(* Logix 5000 Rung export; software revision 13.03 *)

TYPE BIS_M_Userparameter :
STRUCT
   CRC_16 : SINT;   // 00h=disable, 01h=enable
   Simultan : SINT;   // 00h=disable, 01h=enable
   Dynamic_Head1 : SINT;   // 00h=disable, 01h=enable
   Dynamic_Head2 : SINT;   // 00h=disable, 01h=enable
   Extra_Haed1 : SINT;   // 00h=disable, 01h=enable
   Extra_Head2 : SINT;   // 00h=disable, 01h=enable
   Extra_Adr_Head1 : INT;   // 0 - 8191
   Extra_Adr_Head2 : INT;   // 0 - 8191
   TypSN : SINT;   // 00h=disable, 01h=enable
   DTTyp : SINT;   // 00h=All types, 01h=BIS M-1xx, 02h=not valid, 03h=not valid
END_STRUCT
END_TYPE

VAR_GLOBAL   (* controller tags *)
   control_bism1_par3 : MESSAGE;   // Parameter 3 write - Dynamic1
        MessageParameters(MessageType := CIP Generic, RequestedLength := 1, ConnectedFlag := 2, ConnectionPath := BIS_M, ServiceCode := 16#0010, ObjectType := 16#0064, TargetObject := 1, AttributeNumber := 16#0003, LocalElement := Userparameter_write_BISM_1.Dynamic_Head1)
   state_bism1_par1 : MESSAGE;   // Parameter 1 read - CRC
        MessageParameters(MessageType := CIP Generic, ConnectedFlag := 2, ConnectionPath := BIS_M, ServiceCode := 16#000e, ObjectType := 16#0064, TargetObject := 1, AttributeNumber := 16#0001, DestinationTag := Userparameter_read_BISM_1.CRC_16)
   control_bism1_par2 : MESSAGE;   // Parameter 2 write - Simultan
        MessageParameters(MessageType := CIP Generic, RequestedLength := 1, ConnectedFlag := 2, ConnectionPath := BIS_M, ServiceCode := 16#0010, ObjectType := 16#0064, TargetObject := 1, AttributeNumber := 16#0002, LocalElement := Userparameter_write_BISM_1.Simultan)
   control_bism1_par4 : MESSAGE;   // Parameter 4 write - Dynamic2
        MessageParameters(MessageType := CIP Generic, RequestedLength := 1, ConnectedFlag := 2, ConnectionPath := BIS_M, ServiceCode := 16#0010, ObjectType := 16#0064, TargetObject := 1, AttributeNumber := 16#0004, LocalElement := Userparameter_write_BISM_1.Dynamic_Head2)
   control_bism1_par6 : MESSAGE;   // Parameter 6 write - Extra2
        MessageParameters(MessageType := CIP Generic, RequestedLength := 1, ConnectedFlag := 2, ConnectionPath := BIS_M, ServiceCode := 16#0010, ObjectType := 16#0064, TargetObject := 1, AttributeNumber := 16#0006, LocalElement := Userparameter_write_BISM_1.Extra_Head2)
   state_bism1_par4 : MESSAGE;   // Patameter 4 read - Dynamic2
        MessageParameters(MessageType := CIP Generic, ConnectedFlag := 2, ConnectionPath := BIS_M, ServiceCode := 16#000e, ObjectType := 16#0064, TargetObject := 1, AttributeNumber := 16#0004, DestinationTag := Userparameter_read_BISM_1.Dynamic_Head2)
   control_bism1_par9 : MESSAGE;   // Parameter 9 write - Typ SN
        MessageParameters(MessageType := CIP Generic, RequestedLength := 1, ConnectedFlag := 2, ConnectionPath := BIS_M, ServiceCode := 16#0010, ObjectType := 16#0064, TargetObject := 1, AttributeNumber := 16#0009, LocalElement := Userparameter_write_BISM_1.TypSN)
   state_bism1_parA : MESSAGE;   // Patameter 10 read - DTTyp
        MessageParameters(MessageType := CIP Generic, ConnectedFlag := 2, ConnectionPath := BIS_M, ServiceCode := 16#000e, ObjectType := 16#0064, TargetObject := 1, AttributeNumber := 16#000a, DestinationTag := Userparameter_read_BISM_1.DTTyp)
   state_bism1_par7 : MESSAGE;   // Patameter 7 read - Extra_Adr1
        MessageParameters(MessageType := CIP Generic, ConnectedFlag := 2, ConnectionPath := BIS_M, ServiceCode := 16#000e, ObjectType := 16#0064, TargetObject := 1, AttributeNumber := 16#0007, DestinationTag := Userparameter_read_BISM_1.Extra_Adr_Head1)
   state_bism1_par6 : MESSAGE;   // Patameter 6 read - Extra2
        MessageParameters(MessageType := CIP Generic, ConnectedFlag := 2, ConnectionPath := BIS_M, ServiceCode := 16#000e, ObjectType := 16#0064, TargetObject := 1, AttributeNumber := 16#0006, DestinationTag := Userparameter_read_BISM_1.Extra_Head2)
   control_bism1_par1 : MESSAGE;   // Parameter 1write - CRC
        MessageParameters(MessageType := CIP Generic, RequestedLength := 1, ConnectedFlag := 2, ConnectionPath := BIS_M, ServiceCode := 16#0010, ObjectType := 16#0064, TargetObject := 1, AttributeNumber := 16#0001, LocalElement := Userparameter_write_BISM_1.CRC_16)
   Userparameter_read_BISM_1 : BIS_M_Userparameter;
   state_bism1_par3 : MESSAGE;   // Parameter 3 read - Dynamic1
        MessageParameters(MessageType := CIP Generic, ConnectedFlag := 2, ConnectionPath := BIS_M, ServiceCode := 16#000e, ObjectType := 16#0064, TargetObject := 1, AttributeNumber := 16#0003, DestinationTag := Userparameter_read_BISM_1.Dynamic_Head1)
   state_bism1_par2 : MESSAGE;   // Parameter 2 read - Simultan
        MessageParameters(MessageType := CIP Generic, ConnectedFlag := 2, ConnectionPath := BIS_M, ServiceCode := 16#000e, ObjectType := 16#0064, TargetObject := 1, AttributeNumber := 16#0002, DestinationTag := Userparameter_read_BISM_1.Simultan)
   Userparameter_write_BISM_1 : BIS_M_Userparameter;
   state_bism1_par5 : MESSAGE;   // Patameter 5 read - Extra1
        MessageParameters(MessageType := CIP Generic, ConnectedFlag := 2, ConnectionPath := BIS_M, ServiceCode := 16#000e, ObjectType := 16#0064, TargetObject := 1, AttributeNumber := 16#0005, DestinationTag := Userparameter_read_BISM_1.Extra_Haed1)
   control_bism1_par5 : MESSAGE;   // Parameter 5 write - Extra1
        MessageParameters(MessageType := CIP Generic, RequestedLength := 1, ConnectedFlag := 2, ConnectionPath := BIS_M, ServiceCode := 16#0010, ObjectType := 16#0064, TargetObject := 1, AttributeNumber := 16#0005, LocalElement := Userparameter_write_BISM_1.Extra_Haed1)
   control_bism1_parA : MESSAGE;   // Parameter 10 write - DTTyp
        MessageParameters(MessageType := CIP Generic, RequestedLength := 1, ConnectedFlag := 2, ConnectionPath := BIS_M, ServiceCode := 16#0010, ObjectType := 16#0064, TargetObject := 1, AttributeNumber := 16#000a, LocalElement := Userparameter_write_BISM_1.DTTyp)
   control_bism1_par7 : MESSAGE;   // Parameter 7 write - Extra_Adr1
        MessageParameters(MessageType := CIP Generic, RequestedLength := 2, ConnectedFlag := 2, ConnectionPath := BIS_M, ServiceCode := 16#0010, ObjectType := 16#0064, TargetObject := 1, AttributeNumber := 16#0007, LocalElement := Userparameter_write_BISM_1.Extra_Adr_Head1)
   control_bism1_par8 : MESSAGE;   // Parameter 8 write - Extra_Adr2
        MessageParameters(MessageType := CIP Generic, RequestedLength := 2, ConnectedFlag := 2, ConnectionPath := BIS_M, ServiceCode := 16#0010, ObjectType := 16#0064, TargetObject := 1, AttributeNumber := 16#0008, LocalElement := Userparameter_write_BISM_1.Extra_Adr_Head2)
   state_bism1_par9 : MESSAGE;   // Patameter 9 read - TypSN
        MessageParameters(MessageType := CIP Generic, ConnectedFlag := 2, ConnectionPath := BIS_M, ServiceCode := 16#000e, ObjectType := 16#0064, TargetObject := 1, AttributeNumber := 16#0009, DestinationTag := Userparameter_read_BISM_1.TypSN)
   state_bism1_par8 : MESSAGE;   // Patameter 8 read - Extra_Adr2
        MessageParameters(MessageType := CIP Generic, ConnectedFlag := 2, ConnectionPath := BIS_M, ServiceCode := 16#000e, ObjectType := 16#0064, TargetObject := 1, AttributeNumber := 16#0008, DestinationTag := Userparameter_read_BISM_1.Extra_Adr_Head2)
END_VAR

PROGRAM MainProgram
VAR
   Userparameter_Bool : BOOL[32];
END_VAR

ROUTINE Userparameter_BIS_Ethernet_IP   (* ladder *)
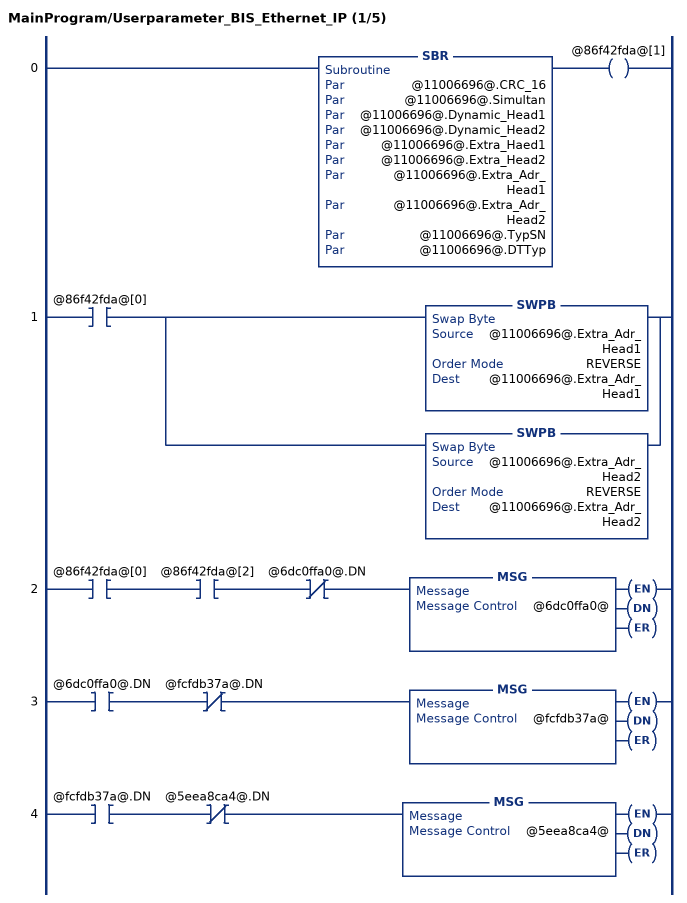
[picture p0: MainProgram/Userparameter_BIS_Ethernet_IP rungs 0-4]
   0: SBR(@11006696@.CRC_16,@11006696@.Simultan,@11006696@.Dynamic_Head1,@11006696@.Dynamic_Head2,@11006696@.Extra_Haed1,@11006696@.Extra_Head2,@11006696@.Extra_Adr_Head1,@11006696@.Extra_Adr_Head2,@11006696@.TypSN,@11006696@.DTTyp)OTE(@86f42fda@[1]);
   1: XIC(@86f42fda@[0])[SWPB(@11006696@.Extra_Adr_Head1,REVERSE,@11006696@.Extra_Adr_Head1) ,SWPB(@11006696@.Extra_Adr_Head2,REVERSE,@11006696@.Extra_Adr_Head2) ];
   2: XIC(@86f42fda@[0])XIC(@86f42fda@[2])XIO(@6dc0ffa0@.DN)MSG(@6dc0ffa0@);
   3: XIC(@6dc0ffa0@.DN)XIO(@fcfdb37a@.DN)MSG(@fcfdb37a@);
   4: XIC(@fcfdb37a@.DN)XIO(@5eea8ca4@.DN)MSG(@5eea8ca4@);
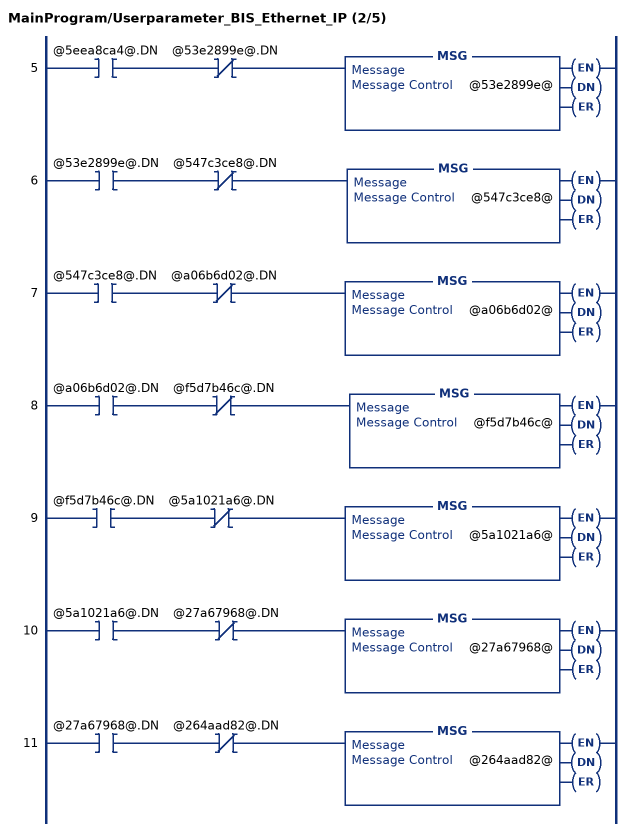
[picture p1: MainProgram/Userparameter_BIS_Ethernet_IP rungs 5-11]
   5: XIC(@5eea8ca4@.DN)XIO(@53e2899e@.DN)MSG(@53e2899e@);
   6: XIC(@53e2899e@.DN)XIO(@547c3ce8@.DN)MSG(@547c3ce8@);
   7: XIC(@547c3ce8@.DN)XIO(@a06b6d02@.DN)MSG(@a06b6d02@);
   8: XIC(@a06b6d02@.DN)XIO(@f5d7b46c@.DN)MSG(@f5d7b46c@);
   9: XIC(@f5d7b46c@.DN)XIO(@5a1021a6@.DN)MSG(@5a1021a6@);
   10: XIC(@5a1021a6@.DN)XIO(@27a67968@.DN)MSG(@27a67968@);
   11: XIC(@27a67968@.DN)XIO(@264aad82@.DN)MSG(@264aad82@);
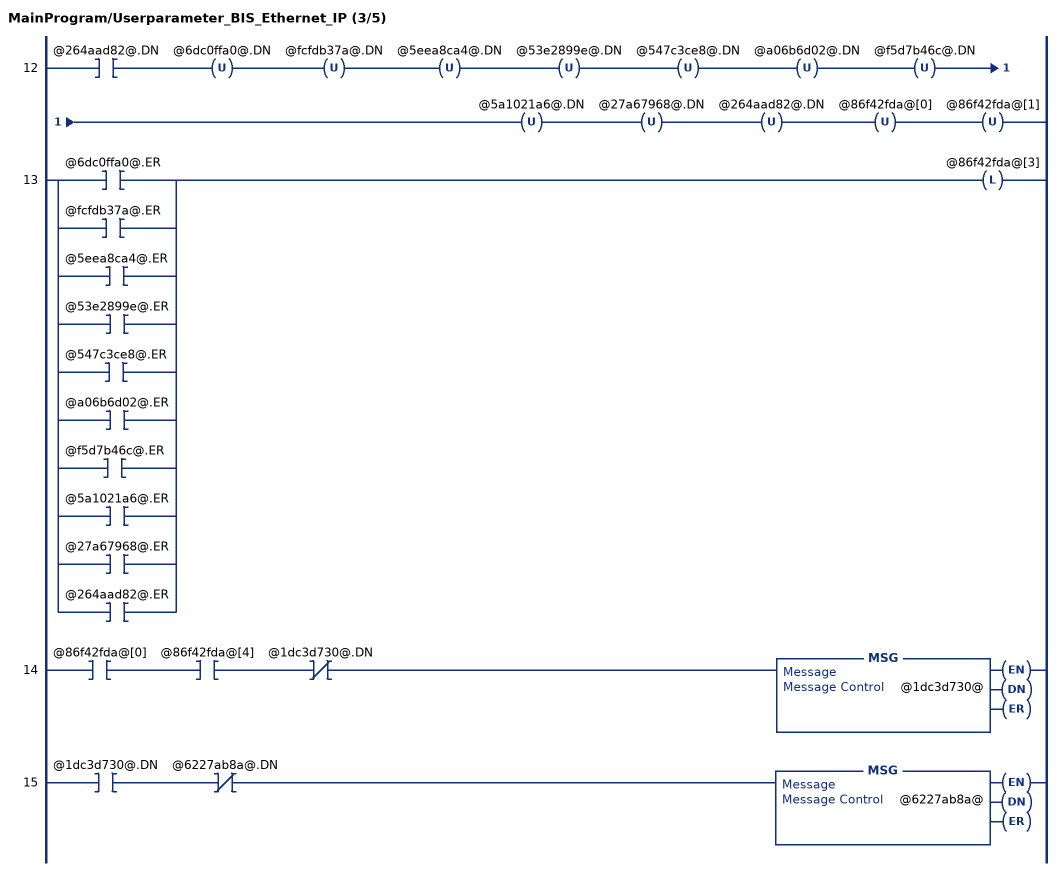
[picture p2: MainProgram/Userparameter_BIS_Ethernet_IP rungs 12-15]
   12: XIC(@264aad82@.DN)OTU(@6dc0ffa0@.DN)OTU(@fcfdb37a@.DN)OTU(@5eea8ca4@.DN)OTU(@53e2899e@.DN)OTU(@547c3ce8@.DN)OTU(@a06b6d02@.DN)OTU(@f5d7b46c@.DN)OTU(@5a1021a6@.DN)OTU(@27a67968@.DN)OTU(@264aad82@.DN)OTU(@86f42fda@[0])OTU(@86f42fda@[1]);
   13: [XIC(@6dc0ffa0@.ER) ,XIC(@fcfdb37a@.ER) ,XIC(@5eea8ca4@.ER) ,XIC(@53e2899e@.ER) ,XIC(@547c3ce8@.ER) ,XIC(@a06b6d02@.ER) ,XIC(@f5d7b46c@.ER) ,XIC(@5a1021a6@.ER) ,XIC(@27a67968@.ER) ,XIC(@264aad82@.ER) ]OTL(@86f42fda@[3]);
   14: XIC(@86f42fda@[0])XIC(@86f42fda@[4])XIO(@1dc3d730@.DN)MSG(@1dc3d730@);
   15: XIC(@1dc3d730@.DN)XIO(@6227ab8a@.DN)MSG(@6227ab8a@);
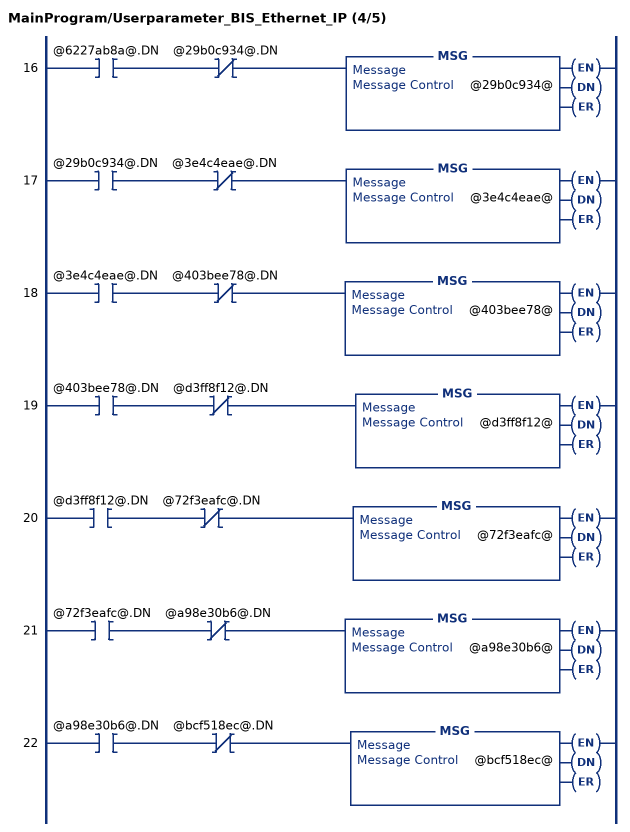
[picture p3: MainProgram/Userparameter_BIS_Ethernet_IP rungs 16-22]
   16: XIC(@6227ab8a@.DN)XIO(@29b0c934@.DN)MSG(@29b0c934@);
   17: XIC(@29b0c934@.DN)XIO(@3e4c4eae@.DN)MSG(@3e4c4eae@);
   18: XIC(@3e4c4eae@.DN)XIO(@403bee78@.DN)MSG(@403bee78@);
   19: XIC(@403bee78@.DN)XIO(@d3ff8f12@.DN)MSG(@d3ff8f12@);
   20: XIC(@d3ff8f12@.DN)XIO(@72f3eafc@.DN)MSG(@72f3eafc@);
   21: XIC(@72f3eafc@.DN)XIO(@a98e30b6@.DN)MSG(@a98e30b6@);
   22: XIC(@a98e30b6@.DN)XIO(@bcf518ec@.DN)MSG(@bcf518ec@);
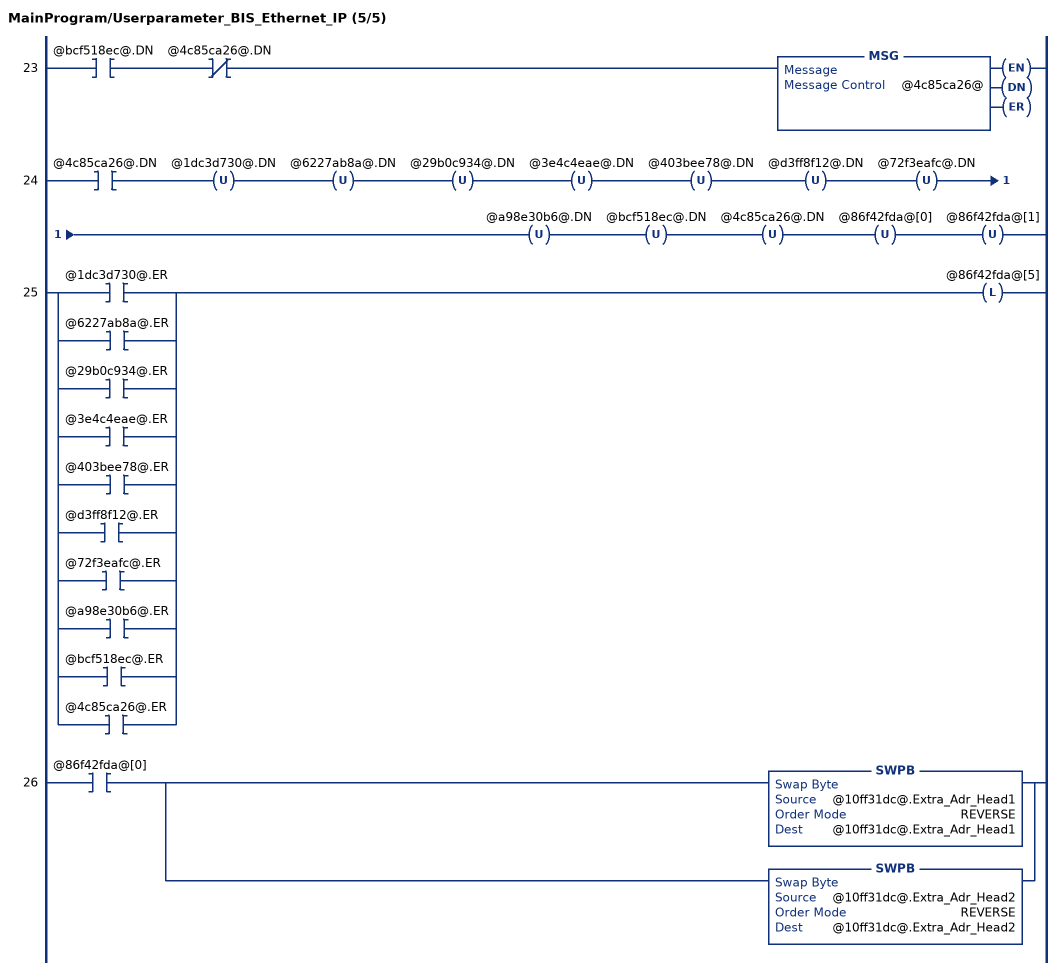
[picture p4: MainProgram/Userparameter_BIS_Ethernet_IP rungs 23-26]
   23: XIC(@bcf518ec@.DN)XIO(@4c85ca26@.DN)MSG(@4c85ca26@);
   24: XIC(@4c85ca26@.DN)OTU(@1dc3d730@.DN)OTU(@6227ab8a@.DN)OTU(@29b0c934@.DN)OTU(@3e4c4eae@.DN)OTU(@403bee78@.DN)OTU(@d3ff8f12@.DN)OTU(@72f3eafc@.DN)OTU(@a98e30b6@.DN)OTU(@bcf518ec@.DN)OTU(@4c85ca26@.DN)OTU(@86f42fda@[0])OTU(@86f42fda@[1]);
   25: [XIC(@1dc3d730@.ER) ,XIC(@6227ab8a@.ER) ,XIC(@29b0c934@.ER) ,XIC(@3e4c4eae@.ER) ,XIC(@403bee78@.ER) ,XIC(@d3ff8f12@.ER) ,XIC(@72f3eafc@.ER) ,XIC(@a98e30b6@.ER) ,XIC(@bcf518ec@.ER) ,XIC(@4c85ca26@.ER) ]OTL(@86f42fda@[5]);
   26: XIC(@86f42fda@[0])[SWPB(@10ff31dc@.Extra_Adr_Head1,REVERSE,@10ff31dc@.Extra_Adr_Head1) ,SWPB(@10ff31dc@.Extra_Adr_Head2,REVERSE,@10ff31dc@.Extra_Adr_Head2) ];
END_ROUTINE
END_PROGRAM
